PROGRAM MAIN

VAR CONSTANT	
    cInitSource1		: ST_MA_MultiArray_InitPars := (eTypeCode := eMA_TypeCode_LREAL, nDims := 1, aDimSizes := [cBufferLength1]);
	cInitSource2		: ST_MA_MultiArray_InitPars := (eTypeCode := eMA_TypeCode_LREAL, nDims := 1, aDimSizes := [cBufferLength2]);	
	cInitSource3		: ST_MA_MultiArray_InitPars := (eTypeCode := eMA_TypeCode_LREAL, nDims := 1, aDimSizes := [cBufferLength3]);
	cInitSource4		: ST_MA_MultiArray_InitPars := (eTypeCode := eMA_TypeCode_LREAL, nDims := 1, aDimSizes := [cBufferLength4]);
	cInitSource5		: ST_MA_MultiArray_InitPars := (eTypeCode := eMA_TypeCode_LREAL, nDims := 1, aDimSizes := [cBufferLength5]);
	cInitSource6		: ST_MA_MultiArray_InitPars := (eTypeCode := eMA_TypeCode_LREAL, nDims := 1, aDimSizes := [cBufferLength6]);	
END_VAR

VAR
	nInputSelection		: UDINT := 1;							// Switch between hardware and function generator	
	nSample				: UDINT;                            	
	aEl3632 AT %I*		: ARRAY[1..cOversamples] OF INT;		// Input from hardware e.g. EL3632
	aBuffer				: ARRAY[1..cOversamples] OF LREAL;  	// signal 
        
	fbFunctionGenerator	: FB_FunctionGenerator;					// Signal Generator
	fSetFrequency		: LREAL := 500.0;						// Hz
	fSetAmplitude		: LREAL := 13.0;						// peak amplitude of sin signal
	
	fbSource1			: FB_CMA_Source :=(stInitPars := cInitSource1, nOwnID := eID_Source1, aDestIDs := [eID_Spectrum1], nResultBuffers := 4);		// Initialize source buffers
	fbSource2			: FB_CMA_Source :=(stInitPars := cInitSource2, nOwnID := eID_Source2, aDestIDs := [eID_Spectrum2], nResultBuffers := 4);		// Initialize source buffers
	fbSource3			: FB_CMA_Source :=(stInitPars := cInitSource3, nOwnID := eID_Source3, aDestIDs := [eID_Spectrum3], nResultBuffers := 4);		// Initialize source buffers
	fbSource4			: FB_CMA_Source :=(stInitPars := cInitSource4, nOwnID := eID_Source4, aDestIDs := [eID_Spectrum4], nResultBuffers := 4);		// Initialize source buffers
	fbSource5			: FB_CMA_Source :=(stInitPars := cInitSource5, nOwnID := eID_Source5, aDestIDs := [eID_Spectrum5], nResultBuffers := 6);		// Initialize source buffers
	fbSource6			: FB_CMA_Source :=(stInitPars := cInitSource6, nOwnID := eID_Source6, aDestIDs := [eID_Spectrum6], nResultBuffers := 8);		// Initialize source buffers
	
	fbSink1				: FB_CMA_Sink := (nOwnID := eID_Sink1);	// Sink result
	fbSink2				: FB_CMA_Sink := (nOwnID := eID_Sink2);	// Sink result
	fbSink3				: FB_CMA_Sink := (nOwnID := eID_Sink3);	// Sink result
	fbSink4				: FB_CMA_Sink := (nOwnID := eID_Sink4);	// Sink result
	fbSink5				: FB_CMA_Sink := (nOwnID := eID_Sink5);	// Sink result
	fbSink6				: FB_CMA_Sink := (nOwnID := eID_Sink6);	// Sink result
	
	aSpectrumResult1	: ARRAY[1..cFFTResult] OF LREAL;		// Copy result
	aSpectrumResult2	: ARRAY[1..cFFTResult] OF LREAL;		// Copy result
	aSpectrumResult3	: ARRAY[1..cFFTResult] OF LREAL;		// Copy result
	aSpectrumResult4	: ARRAY[1..cFFTResult] OF LREAL;		// Copy result
	aSpectrumResult5	: ARRAY[1..cFFTResult] OF LREAL;		// Copy result
	aSpectrumResult6	: ARRAY[1..cFFTResult] OF LREAL;		// Copy result
	
	bCalculate			: BOOL;
	
	fbErrHist			: FB_HRErrHist;							// error monitoring
	
END_VAR

(* Signal input/generation *)

CASE nInputSelection OF
	0:  (* input from EL3632 *)
		FOR nSample := 1 TO cOversamples DO
			aBuffer[nSample] := INT_TO_LREAL(aEl3632[nSample]);
		END_FOR
	1:  (* signal generator *)		
		fbFunctionGenerator(	fFrequency 	:= fSetFrequency,
								fAmplitude 	:= fSetAmplitude,
								eFunction 	:= E_FunctionType.Sine,
								aSignal		:= aBuffer);
END_CASE					

(* Call source to collect data *)

// Window 1
fbSource1.Input1DStd( pDataIn 			:= ADR(aBuffer),
					  nDataInSize 		:= SIZEOF(aBuffer), 
					  eElementType 		:= eMA_TypeCode_LREAL,
					  nOptionPars		:= cCMA_Option_MarkInterruption ); 
IF fbSource1.bError THEN
	fbErrHist.AddError(bErr:=TRUE, hrErrCode:=fbSource1.hrErrorCode, sErrSource:='MAIN.fbSource1'); // error monitoring
	// ToDo: if error
END_IF

// Window 2
fbSource2.Input1DStd( pDataIn 			:= ADR(aBuffer),
					  nDataInSize 		:= SIZEOF(aBuffer), 
					  eElementType 		:= eMA_TypeCode_LREAL,
					  nOptionPars		:= cCMA_Option_MarkInterruption ); 
IF fbSource2.bError THEN
	fbErrHist.AddError(bErr:=TRUE, hrErrCode:=fbSource2.hrErrorCode, sErrSource:='MAIN.fbSource2'); // error monitoring
	// ToDo: if error
END_IF

// Window 3
fbSource3.Input1DStd( pDataIn 			:= ADR(aBuffer),
					  nDataInSize 		:= SIZEOF(aBuffer), 
					  eElementType 		:= eMA_TypeCode_LREAL,
					  nOptionPars		:= cCMA_Option_MarkInterruption ); 
IF fbSource3.bError THEN
	fbErrHist.AddError(bErr:=TRUE, hrErrCode:=fbSource3.hrErrorCode, sErrSource:='MAIN.fbSource3'); // error monitoring
	// ToDo: if error
END_IF

// Window 4
fbSource4.Input1DStd( pDataIn 			:= ADR(aBuffer),
					  nDataInSize 		:= SIZEOF(aBuffer), 
					  eElementType 		:= eMA_TypeCode_LREAL,
					  nOptionPars		:= cCMA_Option_MarkInterruption ); 
IF fbSource4.bError THEN
	fbErrHist.AddError(bErr:=TRUE, hrErrCode:=fbSource4.hrErrorCode, sErrSource:='MAIN.fbSource4'); // error monitoring
	// ToDo: if error
END_IF

// Window 5
fbSource5.Input1DStd( pDataIn 			:= ADR(aBuffer),
					  nDataInSize 		:= SIZEOF(aBuffer), 
					  eElementType 		:= eMA_TypeCode_LREAL,
					  nOptionPars		:= cCMA_Option_MarkInterruption ); 
IF fbSource5.bError THEN
	fbErrHist.AddError(bErr:=TRUE, hrErrCode:=fbSource5.hrErrorCode, sErrSource:='MAIN.fbSource5'); // error monitoring
	// ToDo: if error
END_IF

// Window 6
fbSource6.Input1DStd( pDataIn 			:= ADR(aBuffer),
					  nDataInSize 		:= SIZEOF(aBuffer), 
					  eElementType 		:= eMA_TypeCode_LREAL,
					  nOptionPars		:= cCMA_Option_MarkInterruption ); 
IF fbSource6.bError THEN
	fbErrHist.AddError(bErr:=TRUE, hrErrCode:=fbSource6.hrErrorCode, sErrSource:='MAIN.fbSource6'); // error monitoring
	// ToDo: if error
END_IF

(* Push results to sink *)

// Window 1
fbSink1.Output1DStd(	pDataOut 		:= ADR(aSpectrumResult1), 
						nDataOutSize 	:= SIZEOF(aSpectrumResult1), 
						eElementType 	:= eMA_TypeCode_LREAL, 
						nOptionPars		:= 0,
						bNewResult		=> bCalculate );
IF fbSink1.bError THEN
	fbErrHist.AddError(bErr:=TRUE, hrErrCode:=fbSink1.hrErrorCode, sErrSource:='MAIN.fbSink1'); // error monitoring
	// ToDo: if error
END_IF

// Window 2
fbSink2.Output1DStd(	pDataOut 		:= ADR(aSpectrumResult2), 
						nDataOutSize 	:= SIZEOF(aSpectrumResult2), 
						eElementType 	:= eMA_TypeCode_LREAL, 
						nOptionPars		:= 0,
						bNewResult		=> bCalculate );
IF fbSink2.bError THEN
	fbErrHist.AddError(bErr:=TRUE, hrErrCode:=fbSink2.hrErrorCode, sErrSource:='MAIN.fbSink2'); // error monitoring
	// ToDo: if error
END_IF

// Window 3
fbSink3.Output1DStd(	pDataOut 		:= ADR(aSpectrumResult3), 
						nDataOutSize 	:= SIZEOF(aSpectrumResult3), 
						eElementType 	:= eMA_TypeCode_LREAL, 
						nOptionPars		:= 0,
						bNewResult		=> bCalculate );
IF fbSink3.bError THEN
	fbErrHist.AddError(bErr:=TRUE, hrErrCode:=fbSink3.hrErrorCode, sErrSource:='MAIN.fbSink3'); // error monitoring
	// ToDo: if error
END_IF

// Window 4
fbSink4.Output1DStd(	pDataOut 		:= ADR(aSpectrumResult4), 
						nDataOutSize 	:= SIZEOF(aSpectrumResult4), 
						eElementType 	:= eMA_TypeCode_LREAL, 
						nOptionPars		:= 0,
						bNewResult		=> bCalculate );
IF fbSink4.bError THEN
	fbErrHist.AddError(bErr:=TRUE, hrErrCode:=fbSink4.hrErrorCode, sErrSource:='MAIN.fbSink4'); // error monitoring
	// ToDo: if error
END_IF

// Window 5
fbSink5.Output1DStd(	pDataOut 		:= ADR(aSpectrumResult5), 
						nDataOutSize 	:= SIZEOF(aSpectrumResult5), 
						eElementType 	:= eMA_TypeCode_LREAL, 
						nOptionPars		:= 0,
						bNewResult		=> bCalculate );
IF fbSink5.bError THEN
	fbErrHist.AddError(bErr:=TRUE, hrErrCode:=fbSink5.hrErrorCode, sErrSource:='MAIN.fbSink5'); // error monitoring
	// ToDo: if error
END_IF

// Window 6
fbSink6.Output1DStd(	pDataOut 		:= ADR(aSpectrumResult6), 
						nDataOutSize 	:= SIZEOF(aSpectrumResult6), 
						eElementType 	:= eMA_TypeCode_LREAL, 
						nOptionPars		:= 0,
						bNewResult		=> bCalculate );
IF fbSink6.bError THEN
	fbErrHist.AddError(bErr:=TRUE, hrErrCode:=fbSink6.hrErrorCode, sErrSource:='MAIN.fbSink6'); // error monitoring
	// ToDo: if error
END_IF

END_PROGRAM
